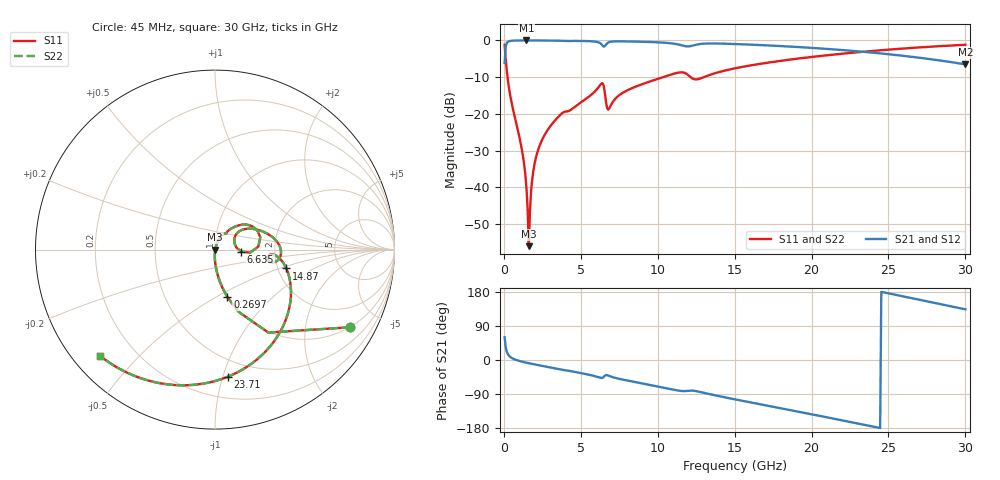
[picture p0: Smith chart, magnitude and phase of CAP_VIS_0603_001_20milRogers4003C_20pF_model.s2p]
! S-parameter model data by Modelithics Inc.  support@modelithics.com  813-866-6335  Tampa FL USA
! S-Parameter data specifications:
! Substrate: 20-mil Rogers 4003C, substrate thickness, H=0.508mm, Dielectric constant, Er=3.75
! PCB Mounting Pad Footprint: Pad width, PadW=0.90mm , Pad length, PadL=1.00mm , Pad gap, PadG (edge-to-edge)=1.00mm , Reference planes=3.0mm apart
! Created Wed Nov 18 13:27:12 2015
# hz S ma R 50
! 2 Port Network Data from SP1.SP block
! freq  magS11  angS11  magS21  angS21  magS12  angS12  magS22  angS22
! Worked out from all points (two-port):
!   401 points, 45 MHz to 30 GHz, reference 50 ohm
!   highest |S21| = -0.01 dB at 1.468 GHz (marker M1); lowest = -6.5 dB at 30 GHz (marker M2)
!   |S21| within 3 dB of the highest: 96.12 MHz to 23.14 GHz (23.04 GHz wide, 198 % of centre)
!   lowest |S11| = -56.0 dB at 1.618 GHz (marker M3), VSWR 1.00, Z = 50.2 - j0.0247 ohm
!   |S11| at or under -10 dB: 235.1 MHz to 10.35 GHz (10.11 GHz wide, 191 % of centre); 12.14 GHz to 13 GHz (857.7 MHz wide, 6.82 % of centre)
!   |S22| runs from -56.0 to -1.2 dB; largest |S21 - S12| = 0
!   S11 on the Smith chart (normalised r, x): 45 MHz: 0.99, -3.50; 269.7 MHz: 0.99, -0.57; 6.635 GHz: 1.34, -0.03; 14.87 GHz: 2.22, -0.56; 23.71 GHz: 0.36, -1.04; 30 GHz: 0.08, -0.39
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4.5e7  0.8696 -29.8  0.4937 60.2  0.4937 60.2  0.8696 -29.8
2.696625e8  0.2749 -75.3  0.9608 14.5  0.9608 14.5  0.2749 -75.3
1.168312e9  0.03265 -91.9  0.998 -4.3  0.998 -4.3  0.03265 -91.9
1.318088e9  0.0204 -91.7  0.9982 -5.8  0.9982 -5.8  0.0204 -91.7
1.467862e9  0.009748 -88.2  0.9983 -7.2  0.9983 -7.2  0.009748 -88.2
1.617638e9  0.001591 -8.9  0.9983 -8.5  0.9983 -8.5  0.001591 -8.9
1.767412e9  0.008947 69.5  0.9981 -9.8  0.9981 -9.8  0.008947 69.5
1.992075e9  0.02096 73.5  0.9978 -11.7  0.9978 -11.7  0.02096 73.5
2.516288e9  0.04604 71.6  0.9966 -15.9  0.9966 -15.9  0.04604 71.6
3.6396e9  0.09599 62.0  0.9894 -24.6  0.9894 -24.6  0.09599 62.0
5.062462e9  0.1463 52.6  0.9827 -35.0  0.9827 -35.0  0.1463 52.6
6.33555e9  0.2588 24.4  0.8883 -47.5  0.8883 -47.5  0.2588 24.4
6.6351e9  0.1463 -4.4  0.8765 -39.7  0.8765 -39.7  0.1463 -4.4
6.859762e9  0.1202 26.8  0.9505 -42.4  0.9505 -42.4  0.1202 26.8
7.8333e9  0.1997 34.8  0.9701 -52.6  0.9701 -52.6  0.1997 34.8
1.007992e10  0.3033 17.2  0.94 -70.5  0.94 -70.5  0.3033 17.2
1.487272e10  0.411 -14.8  0.8951 -102.7  0.8951 -102.7  0.411 -14.8
1.50225e10  0.4172 -15.9  0.8928 -103.9  0.8928 -103.9  0.4172 -15.9
2.003996e10  0.5966 -54.5  0.7906 -143.5  0.7906 -143.5  0.5966 -54.5
2.370945e10  0.7115 -84.1  0.6896 -173.4  0.6896 -173.4  0.7115 -84.1
2.505742e10  0.7505 -95.3  0.6471 175.4  0.6471 175.4  0.7505 -95.3
3e10  0.8718 -137.0  0.4723 133.7  0.4723 133.7  0.8718 -137.0
